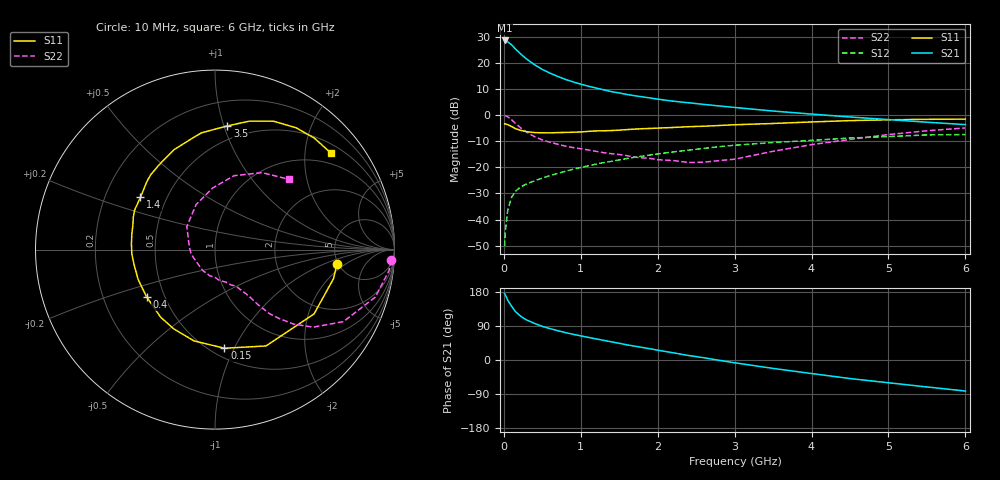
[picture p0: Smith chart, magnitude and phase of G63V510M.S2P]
! SIEMENS Small Signal Semiconductors
! BFG193
! Si NPN RF Bipolar Junction Transistor in SOT223
! VCE = 3.5 V  IC = 10 mA
! Common Emitter S-Parameters:  August  1996
# GHz  S  MA  R  50
!  f  S11  S21  S12  S22
! GHz  MAG  ANG  MAG  ANG  MAG  ANG  MAG  ANG
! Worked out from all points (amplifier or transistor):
!   36 points, 10 MHz to 6 GHz, reference 50 ohm
!   highest |S21| = 28.6 dB at 10 MHz (marker M1)
!   |S21| within 3 dB of that: start of sweep to 142.7 MHz
!   unconditionally stable (mu >= 1): 878.7 MHz to 2.546 GHz
!   at 250 MHz: K = 0.54, MSG = 24.8 dB, |S12| = -27.0 dB
!   at 1.4 GHz: K = 1.07, MAG = 11.7 dB, |S12| = -17.7 dB
!   at 6 GHz: K = 0.87, MSG = 1.9 dB, |S12| = -7.4 dB
!   S11 on the Smith chart (normalised r, x): 10 MHz: 4.86, -1.48; 150 MHz: 0.58, -0.92; 400 MHz: 0.40, -0.27; 1.4 GHz: 0.36, +0.28; 3.5 GHz: 0.39, +1.03; 6 GHz: 0.71, +2.59
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0.01  0.684 -6.8  26.95 175.2  0.0031 92.0  0.9835 -3.4
0.02  0.6797 -13.8  26.75 171.7  0.0061 82.3  0.9767 -6.9
0.05  0.658 -33.0  25.47 158.2  0.0149 75.2  0.9314 -16.5
0.1  0.6074 -62.1  22.25 142.0  0.0267 65.1  0.8202 -29.3
0.15  0.5522 -84.5  18.58 128.0  0.0346 57.4  0.6971 -38.3
0.2  0.5218 -103.0  15.84 118.8  0.0403 53.6  0.6044 -43.4
0.25  0.498 -117.3  13.53 111.1  0.0446 51.3  0.5235 -47.1
0.3  0.4835 -128.7  11.76 105.2  0.0488 50.4  0.469 -49.6
0.4  0.4634 -145.4  9.218 96.5  0.0553 49.7  0.3868 -52.1
0.5  0.4594 -158.8  7.511 88.7  0.0622 49.8  0.3355 -53.4
0.6  0.4585 -169.1  6.381 82.9  0.0695 50.4  0.3031 -54.8
0.7  0.4641 -177.0  5.527 77.3  0.0767 51.1  0.2779 -56.6
0.9  0.4715 169.1  4.338 67.8  0.0922 50.3  0.2395 -59.6
1.1  0.4893 158.5  3.582 59.6  0.1073 49.5  0.2155 -65.8
1.4  0.5075 145.0  2.824 47.9  0.1305 46.2  0.1827 -75.7
1.7  0.5403 133.7  2.354 36.6  0.1561 42.4  0.1572 -88.4
2.2  0.5813 117.6  1.853 19.0  0.1977 33.5  0.1352 -120.5
2.8  0.6342 101.3  1.502 -0.8  0.2492 21.7  0.1349 -170.1
3.5  0.6926 84.3  1.2 -22.2  0.2994 5.8  0.2035 140.5
4.5  0.7862 65.5  0.922 -48.9  0.3651 -14.1  0.3435 92.2
5.5  0.8322 48.2  0.733 -71.1  0.4186 -38.3  0.5023 58.6
6  0.8401 39.9  0.659 -81.9  0.4255 -52.3  0.5699 43.3
